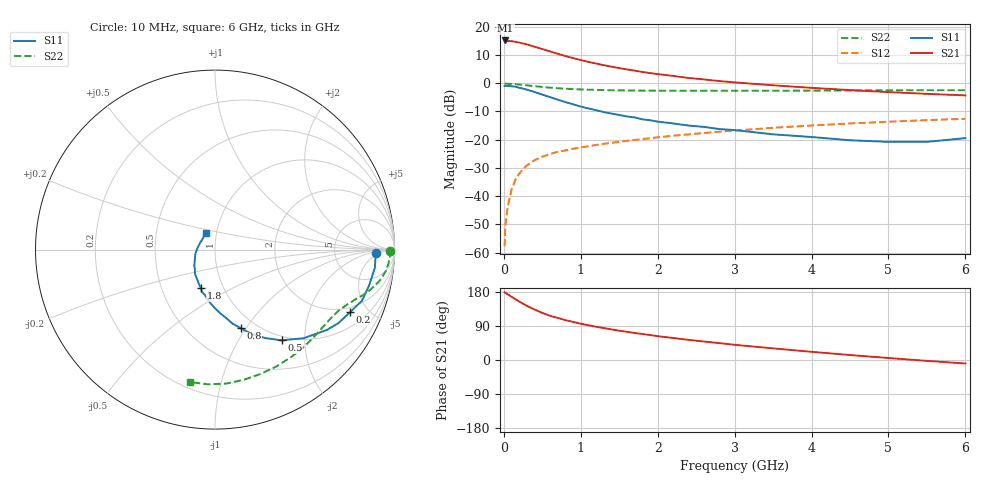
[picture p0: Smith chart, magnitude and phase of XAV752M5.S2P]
! SIEMENS Discrete & RF Semiconductors
! BFY180
! Si NPN RF Bipolar Junction Transistor in MICRO-X
! VCE = 0.75 V  IC = 2.5 mA
! Common Emitter S-Parameters:  May  1997
# GHz  S  MA  R  50
!  f  S11  S21  S12  S22
! GHz  MAG  ANG  MAG  ANG  MAG  ANG  MAG  ANG
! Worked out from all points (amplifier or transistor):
!   36 points, 10 MHz to 6 GHz, reference 50 ohm
!   highest |S21| = 15.1 dB at 20 MHz (marker M1)
!   |S21| within 3 dB of that: start of sweep to 496.2 MHz
!   unconditionally stable (mu >= 1): 879.8 MHz to end of sweep
!   at 250 MHz: K = 0.35, MSG = 22.2 dB, |S12| = -30.4 dB
!   at 1.4 GHz: K = 1.31, MAG = 10.2 dB, |S12| = -21.1 dB
!   at 6 GHz: K = 1.51, MAG = -0.1 dB, |S12| = -12.6 dB
!   S11 on the Smith chart (normalised r, x): 10 MHz: 18, -4; 200 MHz: 1.71, -3.81; 500 MHz: 0.93, -1.55; 800 MHz: 0.85, -0.95; 1.8 GHz: 0.78, -0.36; 6 GHz: 0.89, +0.17
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0.01  0.8977 -1.3  5.599 178.9  0.0013 88.6  0.9753 -0.4
0.02  0.8953 -2.5  5.707 177.2  0.0031 87.2  0.9821 -0.9
0.05  0.8964 -6.5  5.577 173.5  0.0064 83.3  0.9753 -2.4
0.1  0.8819 -13.0  5.549 166.9  0.0131 81.7  0.9692 -4.7
0.15  0.8675 -19.1  5.404 160.5  0.0195 77.1  0.96 -7.0
0.2  0.829 -24.9  5.239 154.3  0.0249 74.2  0.9459 -9.0
0.3  0.7674 -35.7  4.857 142.9  0.0349 67.5  0.9147 -12.5
0.4  0.6982 -45.0  4.418 133.1  0.0434 62.6  0.8857 -15.3
0.5  0.6272 -53.7  4.026 124.2  0.0499 58.7  0.8574 -17.5
0.6  0.5669 -60.4  3.652 116.7  0.0556 56.2  0.8324 -19.3
0.8  0.4617 -71.8  3.014 105.2  0.0646 52.3  0.7979 -22.5
1  0.3848 -80.9  2.573 95.7  0.073 50.1  0.7749 -25.3
1.1  0.3574 -85.1  2.381 91.7  0.0764 49.1  0.7662 -26.6
1.2  0.3317 -89.2  2.225 87.7  0.0807 48.4  0.7599 -28.1
1.4  0.2895 -96.8  1.961 80.7  0.0877 47.4  0.7491 -31.0
1.8  0.229 -110.1  1.581 68.7  0.1023 45.7  0.7384 -36.9
2.2  0.1938 -120.6  1.345 58.1  0.1173 43.2  0.7349 -43.0
2.8  0.154 -136.8  1.09 44.6  0.1383 39.6  0.7336 -52.0
3.5  0.1243 -154.6  0.917 30.7  0.162 34.6  0.7354 -62.4
4.5  0.0976 174.0  0.754 13.1  0.1936 26.5  0.7427 -77.4
5.5  0.0915 138.9  0.647 -2.3  0.2217 17.9  0.7516 -93.0
6  0.1064 118.6  0.608 -9.2  0.2342 13.4  0.7509 -100.8
